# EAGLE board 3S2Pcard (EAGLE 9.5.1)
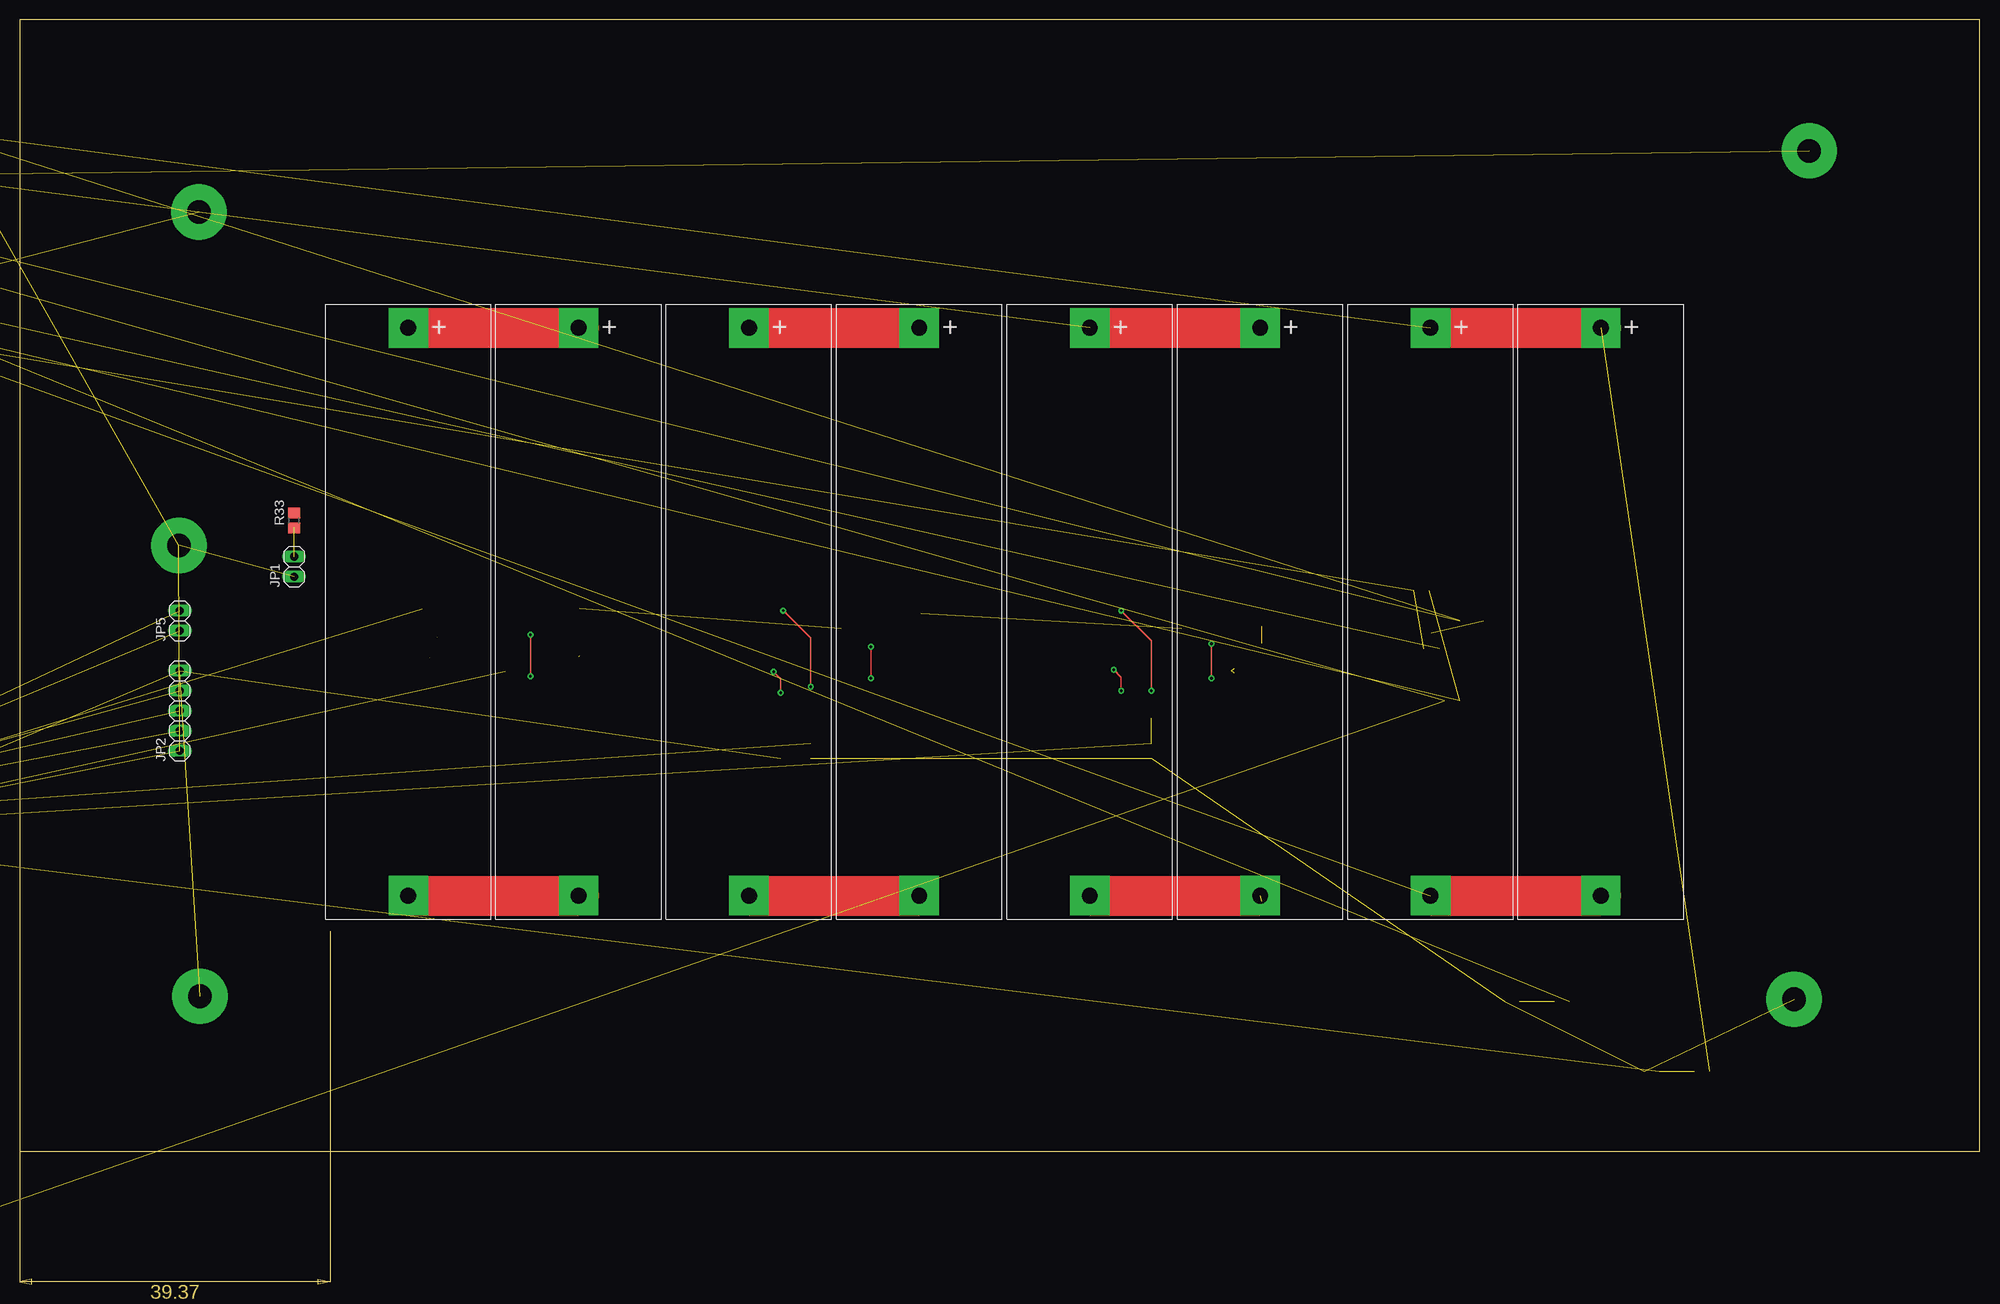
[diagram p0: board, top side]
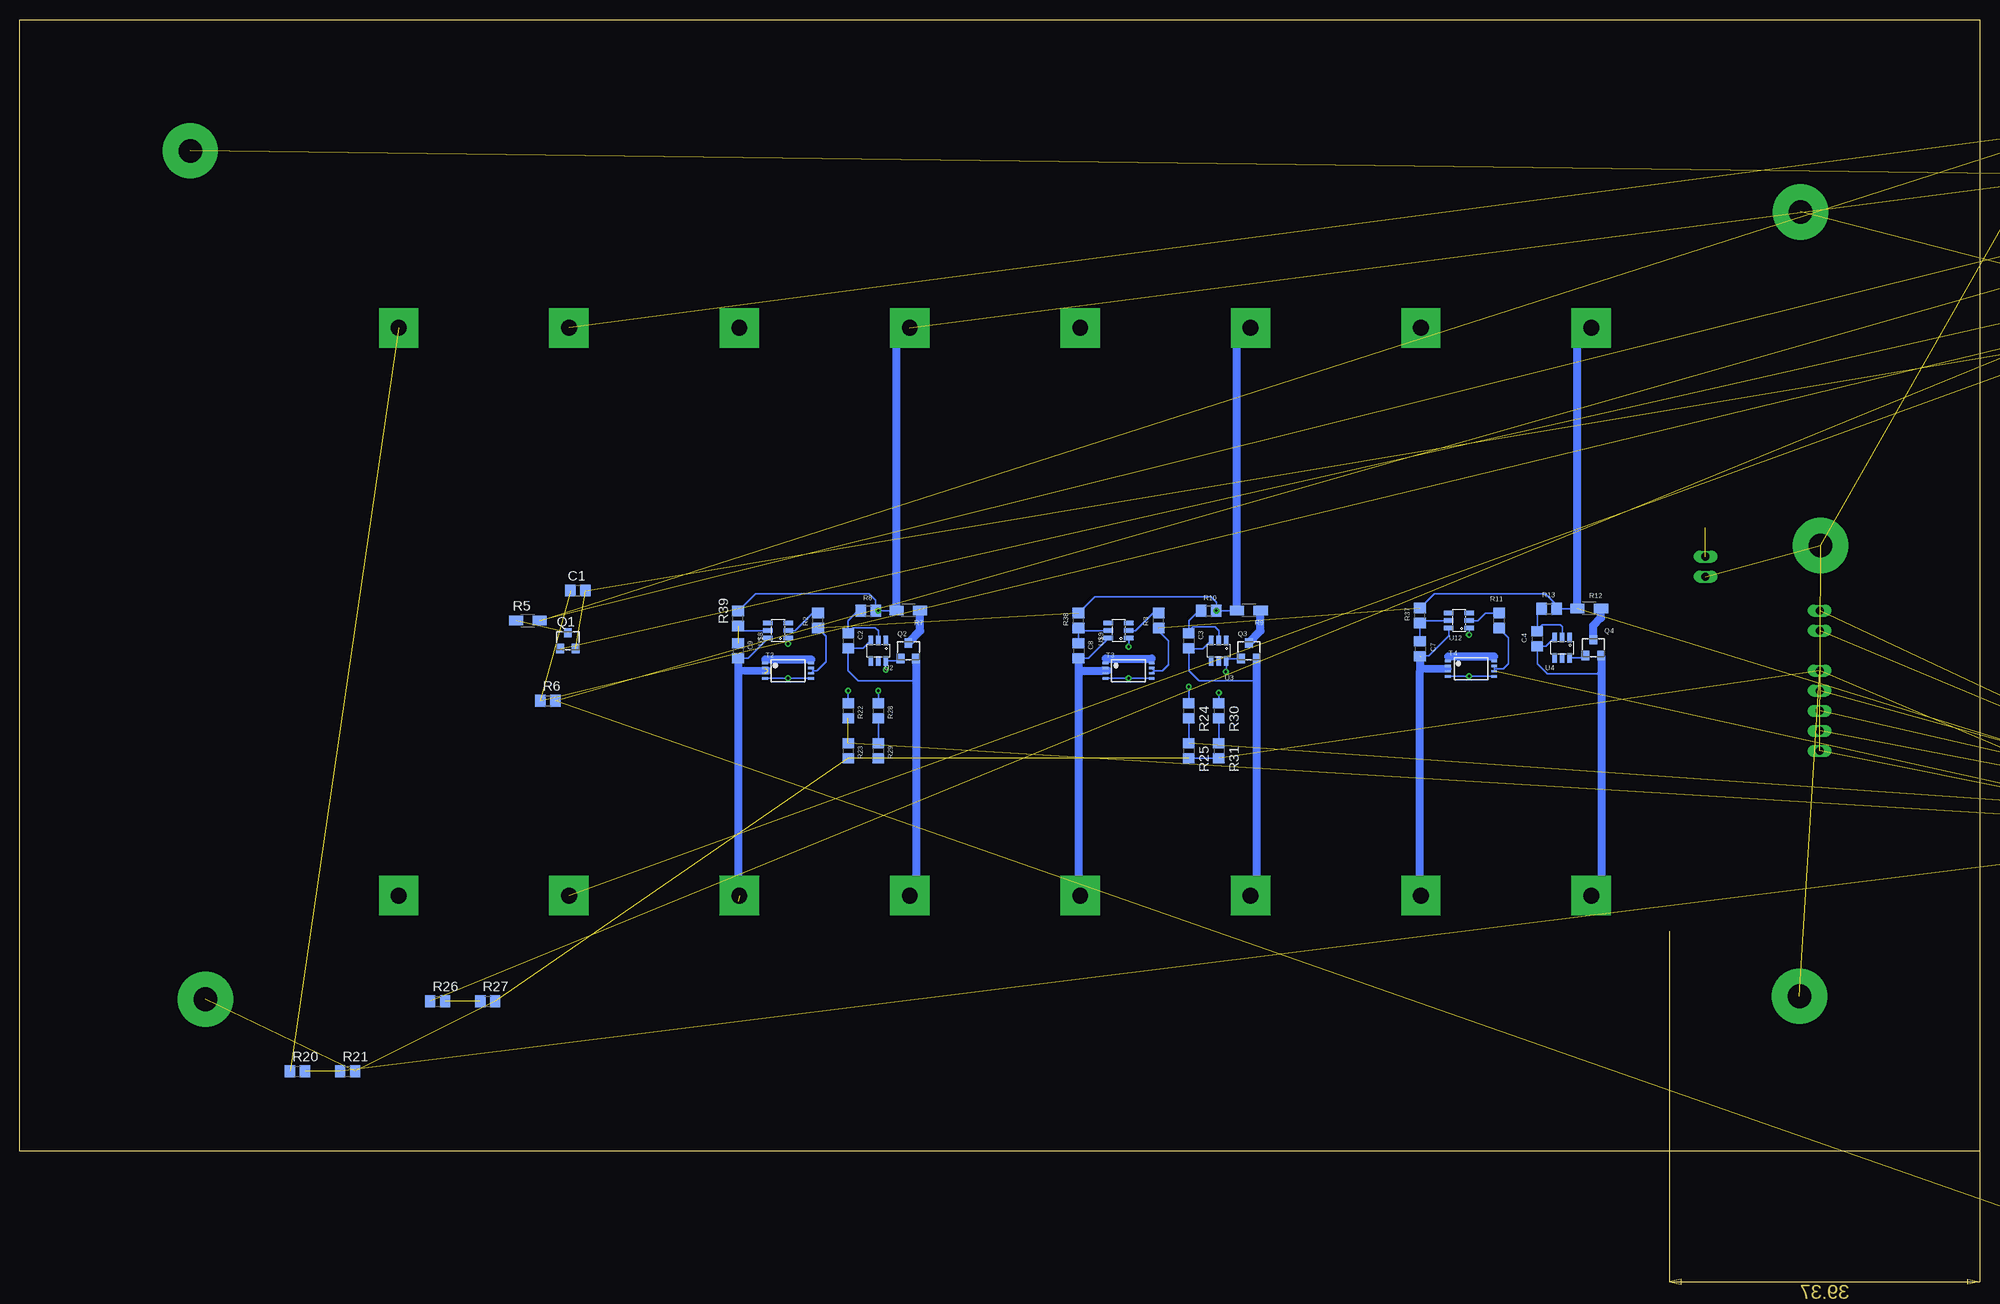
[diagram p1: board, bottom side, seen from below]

Size 248.59 x 160.31 mm. Coordinates in mm from the lower left corner, seen from the top.
Outline: 0,16.81 248.59,16.81 248.59,160.31 0,160.31 0,16.81
Copper layers (1*16): Top 0.035mm / dielectric 1.5mm / Bottom 0.035mm
Design rules "default": minimum track width 6mil, minimum drill 0.35mm, track to track 6mil, track to pad 6mil, pad to pad 6mil, via to via 6mil, smd to smd 6mil, copper to edge 40mil, drill to drill 6mil, minimum pad ring 10mil, minimum via ring 8mil, stop-mask expansion 4mil, vias tented up to drill 0mil, thermal gap 10mil

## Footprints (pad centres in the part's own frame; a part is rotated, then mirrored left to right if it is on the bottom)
18650_HOLDER = drill 2 pad 5 square: + -0.93,38.17; - -0.93,-33.83
C0805 = smd 1.3 x 1.5: 1 -0.95,0; 2 0.95,0
SO08 = smd 0.6 x 2.2: 1 -1.905,-2.6; 2 -0.635,-2.6; 3 0.635,-2.6; 4 1.905,-2.6; 5 1.905,2.6; 6 0.635,2.6; 7 -0.635,2.6; 8 -1.905,2.6
1X02 = drill 1.016 long: 1 -1.27,0; 2 1.27,0
1X05 = drill 1.016 long: 1 -5.08,0; 2 -2.54,0; 3 0,0; 4 2.54,0; 5 5.08,0
0207/10 = drill 0.813 octagon: 1 -5.08,0; 2 5.08,0
CHIP-LED0805 = smd 1.2 x 1.2: A 0,-1.05; C 0,1.05
TO236 = smd 1 x 1.2: 1 0,1; 2 -1,-1; 3 1,-1
SOIC8 = smd 0.6 x 2.2: 1 -1.905,-2.6; 2 -0.635,-2.6; 3 0.635,-2.6; 4 1.905,-2.6; 5 1.905,2.6; 6 0.635,2.6; 7 -0.635,2.6; 8 -1.905,2.6
SOT-23-CBE = smd 1 x 1.4: B -0.95,-1.1; C 0,1.1; E 0.95,-1.1
R0805 = smd 1.3 x 1.5: 1 -0.95,0; 2 0.95,0
R-27X13 = drill 1 square: 1 3.34,6.25; 2 23.66,6.25
R1206W = smd 1.8 x 1.2: 1 -1.499,0; 2 1.499,0
TSSOP-8 = smd 0.3 x 0.75: 1 -0.975,-2.925; 2 -0.325,-2.925; 3 0.325,-2.925; 4 0.975,-2.925; 5 0.975,2.925; 6 0.325,2.925; 7 -0.325,2.925; 8 -0.975,2.925
SOT23-6 = smd 0.55 x 1.2: 1 -0.95,-1.3; 2 0,-1.3; 3 0.95,-1.3; 4 0.95,1.3; 5 0,1.3; 6 -0.95,1.3
QFP80P900X900X120-32N = smd 1.473 x 0.508: 1 -4.242,2.794; 2 -4.242,2.007; 3 -4.242,1.194; 4 -4.242,0.406; 5 -4.242,-0.406; 6 -4.242,-1.194; 7 -4.242,-2.007; 8 -4.242,-2.794; 17 4.242,-2.794; 18 4.242,-2.007; 19 4.242,-1.194; 20 4.242,-0.406; 21 4.242,0.406; 22 4.242,1.194; 23 4.242,2.007; 24 4.242,2.794 | smd 0.508 x 1.473: 9 -2.794,-4.242; 10 -2.007,-4.242; 11 -1.194,-4.242; 12 -0.406,-4.242; 13 0.406,-4.242; 14 1.194,-4.242; 15 2.007,-4.242; 16 2.794,-4.242; 25 2.794,4.242; 26 2.007,4.242; 27 1.194,4.242; 28 0.406,4.242; 29 -0.406,4.242; 30 -1.194,4.242; 31 -2.007,4.242; 32 -2.794,4.242
SPACER = drill 3 pad 7: 1 0,0

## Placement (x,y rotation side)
B11  18650_HOLDER  [18650_HOLDER]  71.81,83.07 0 top
B12  18650_HOLDER  [18650_HOLDER]  50.21,83.07 0 top
B21  18650_HOLDER  [18650_HOLDER]  115.03,83.07 0 top
B22  18650_HOLDER  [18650_HOLDER]  93.42,83.07 0 top
B31  18650_HOLDER  [18650_HOLDER]  158.25,83.07 0 top
B32  18650_HOLDER  [18650_HOLDER]  136.64,83.07 0 top
B41  18650_HOLDER  [18650_HOLDER]  179.85,83.07 0 top
B42  18650_HOLDER  [18650_HOLDER]  201.46,83.07 0 top
C1  [C0805]  177.8,87.93 0 bottom
C2  [C0805]  143.51,81.58 270 bottom
C3  [C0805]  100.33,81.58 270 bottom
C4  [C0805]  56.13,81.83 270 bottom
C5  [C0805]  not placed on the board
C6  [C0805]  not placed on the board
C7  100nF  [C0805]  70.99,80.56 270 bottom
C8  100nF  [C0805]  114.3,80.31 270 bottom
C9  100nF  [C0805]  157.48,80.31 270 bottom
C10  100nF  [C0805]  not placed on the board
IC1  LM358D  [SO08]  not placed on the board
JP1  [1X02]  34.8,90.98 90 top
JP2  [1X05]  20.32,72.69 90 top
JP3  [1X02]  not placed on the board
JP4  [1X02]  not placed on the board
JP5  [1X02]  20.32,84.12 90 top
L1  [0207/10]  not placed on the board
L2  [0207/10]  not placed on the board
L3  [0207/10]  not placed on the board
LED1  RED  [CHIP-LED0805]  not placed on the board
LED2  GREEN  [CHIP-LED0805]  not placed on the board
LED3  BLUE  [CHIP-LED0805]  not placed on the board
Q1  2302  [TO236]  179.07,81.58 0 bottom
Q2  2302  [TO236]  135.89,80.31 0 bottom
Q3  2302  [TO236]  92.71,80.31 0 bottom
Q4  2302  [TO236]  49.02,80.69 0 bottom
Q5  AO4407  [SOIC8]  not placed on the board
Q6  MMBT2222  [SOT-23-CBE]  not placed on the board
Q7  AO4407  [SOIC8]  not placed on the board
Q8  MMBT2222  [SOT-23-CBE]  not placed on the board
R1  1K  [R0805]  not placed on the board
R2  1K  [R0805]  147.32,84.12 90 bottom
R3  1K  [R0805]  104.14,84.12 90 bottom
R4  R-POWER-27X13  [R-27X13]  not placed on the board
R5  [R1206W]  184.15,84.12 0 bottom
R6  [R0805]  181.61,73.96 0 bottom
R7  [R1206W]  135.89,85.39 180 bottom
R8  [R0805]  140.97,85.39 0 bottom
R9  [R1206W]  92.71,85.39 180 bottom
R10  [R0805]  97.79,85.39 0 bottom
R11  1K  [R0805]  60.96,84.12 90 bottom
R12  [R1206W]  49.53,85.64 180 bottom
R13  [R0805]  54.61,85.64 0 bottom
R14  [R0805]  not placed on the board
R15  [R0805]  not placed on the board
R16  [R0805]  not placed on the board
R17  [R0805]  not placed on the board
R18  [R0805]  not placed on the board
R19  [R0805]  not placed on the board
R20  100K  [R0805]  213.36,26.97 0 bottom
R21  470K  [R0805]  207.01,26.97 0 bottom
R22  100K  [R0805]  143.51,72.69 270 bottom
R23  330K  [R0805]  143.51,67.61 270 bottom
R24  100K  [R0805]  100.33,72.69 270 bottom
R25  220K  [R0805]  100.33,67.61 270 bottom
R26  100K  [R0805]  195.58,35.86 0 bottom
R27  470K  [R0805]  189.23,35.86 0 bottom
R28  100K  [R0805]  139.7,72.69 270 bottom
R29  330K  [R0805]  139.7,67.61 270 bottom
R30  100K  [R0805]  96.52,72.69 270 bottom
R31  220K  [R0805]  96.52,67.61 270 bottom
R32  [R0805]  not placed on the board
R33  330K  [R0805]  34.8,96.82 90 top
R34  1K  [R0805]  not placed on the board
R35  1K  [R0805]  not placed on the board
R36  1K  [R0805]  not placed on the board
R37  100E  [R0805]  70.99,84.75 90 bottom
R38  100E  [R0805]  114.3,84.12 90 bottom
R39  100E  [R0805]  157.48,84.37 90 bottom
R40  100E  [R0805]  not placed on the board
T1  DMN3024LSD  [TSSOP-8]  not placed on the board
T2  DMN3024LSD  [TSSOP-8]  151.13,77.77 270 bottom
T3  DMN3024LSD  [TSSOP-8]  107.95,77.77 270 bottom
T4  DMN3024LSD  [TSSOP-8]  64.52,78.02 270 bottom
U1  HY2213  [SOT23-6]  not placed on the board
U2  HY2213  [SOT23-6]  139.7,80.31 180 bottom
U3  HY2213  [SOT23-6]  96.52,80.31 180 bottom
U4  HY2213  [SOT23-6]  52.96,80.69 180 bottom
U5  ATMEGA328P-AU  [QFP80P900X900X120-32N]  not placed on the board
U12  DW01A  [SOT23-6]  66.04,84.12 90 bottom
U$7  DW01A  [SOT23-6]  not placed on the board
U$8  DW01A  [SOT23-6]  152.4,82.85 90 bottom
U$9  DW01A  [SOT23-6]  109.22,82.85 90 bottom
U$13  METAL_SPACER  [SPACER]  226.95,143.68 0 top
U$14  METAL_SPACER  [SPACER]  225.04,36.11 0 top
U$15  METAL_SPACER  [SPACER]  22.73,135.94 0 top
U$16  METAL_SPACER  [SPACER]  22.86,36.5 0 top
U$17  METAL_SPACER  [SPACER]  20.19,93.64 0 top

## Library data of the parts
B11 B12 B21 B22 B31 B32 B41 B42 U$13-U$17 = drag-custom
C1-C10 = rcl; SPICEPREFIX: C
IC1 = linear
JP1-JP5 = pinhead
L1-L3 = rcl; SPICEPREFIX: L
LED1-LED3 = led
Q1-Q8 U1-U4 = drag-semiconductors
R1-R3 R5-R40 = rcl; SPICEPREFIX: R
R4 = drag-rlcd
T1-T4 = FS8205A
U5 = ATmega328-AU; DESCRIPTION: 8-bit Microcontroller with In-System Programmable Flash; MPN: ATMEGA328P-AU; OC_FARNELL: 1715486; OC_NEWARK: 14R4631; PACKAGE: TQFP-32; SUPPLIER: Atmel
U12 U$7-U$9 = DW01A

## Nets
1S+: B11.+ B12.+ R3.1 R12.2 R13.2 R37.2 T3.6 T3.7 U5.26
1S-: B11.- B12.- C4.2 C7.2 Q4.3 T4.2 T4.3 U4.3 U12.6
1S_STATUS: Q4.2 U4.6
2S+: B21.+ B22.+ R2.1 R9.2 R10.2 R24.1 R38.2 T2.6 T2.7
2S-: B21.- B22.- C3.2 C8.2 Q3.3 T3.2 T3.3 U3.3 U$9.6
2S_STATUS: R30.2 R31.1
3S+: B31.+ B32.+ R1.1 R7.2 R8.2 R22.1 R39.2 T1.6 T1.7
3S-: B31.- B32.- C2.2 C9.2 Q2.3 T2.2 T2.3 U2.3 U$8.6
3S_STATUS: R28.2 R29.1
4S+: B41.+ B42.+ JP4.1 L1.2 Q7.5 Q7.6 Q7.7 Q7.8 R5.2 R6.2 R18.2 R20.1 R40.2
4S-: B41.- B42.- C1.2 C10.2 Q1.3 T1.2 T1.3 U1.3 U$7.6
4S_STATUS: R26.2 R27.1
5V: IC1.8 JP1.1 JP2.1 L3.1 LED1.A LED2.A LED3.A R15.2 U5.4 U5.6 U$17.1
ADC_2S: R24.2 R25.1 U5.25
ADC_3S: R22.2 R23.1 U5.24
ADC_4S: R20.2 R21.1 U5.23
BATT_CURR: C5.1 IC1.1 IC1.2 R14.2 R15.1 R32.1 R32.2
CH_SWITCH: R17.2
CHARGE+: JP3.1 Q5.5 Q5.6 Q5.7 Q5.8 R16.2 U$15.1
GND: C5.2 C6.2 IC1.4 JP2.5 Q6.E Q8.E R4.1 R14.1 R21.2 R23.2 R25.2 R27.2 R29.2 R31.2 U5.3 U5.5 U5.21 U$14.1 U$16.1
LOAD+: L2.2 U$13.1
LOAD_SWITCH: R19.2
N$1: C7.1 R37.1 U12.5
N$2: T1.1 T1.8
N$3: C8.1 R38.1 U$9.5
N$5: T2.1 T2.8
N$6: R33.2
N$7: C9.1 R39.1 U$8.5
N$8: C10.1 R40.1 U$7.5
N$9: R1.2 U$7.2
N$10: T1.4 T1.5 U$7.1
N$11: R2.2 U$8.2
N$12: T3.1 T3.8
N$13: C6.1 L3.2 U5.18
N$14: T2.4 T2.5 U$8.1
N$15: LED1.C R34.1
N$16: LED2.C R35.1
N$17: T3.4 T3.5 U$9.1
N$18: R3.2 U$9.2
N$19: LED3.C R36.1
N$20: C1.1 R6.1 U1.2
N$22: Q1.2 R26.1 U1.6
N$23: Q1.1 R5.1
N$25: C2.1 R8.1 U2.2
N$26: Q2.2 R28.1 U2.6
N$27: Q2.1 R7.1
N$28: JP3.2 L1.1 Q5.1 Q5.2 Q5.3
N$30: C3.1 R10.1 U3.2
N$31: Q3.2 R30.1 U3.6
N$32: Q3.1 R9.1
N$33: T4.1 T4.8
N$34: T4.4 T4.5 U12.1
N$36: R11.2 U12.2
N$37: C4.1 R13.1 U4.2
N$38: JP4.2
N$39: Q4.1 R12.1
N$40: IC1.3 R4.2 R11.1 T4.6 T4.7
N$41: Q5.4 Q6.C R16.1
N$42: Q6.B R17.1
N$46: L2.1 Q7.1 Q7.2 Q7.3
N$47: Q7.4 Q8.C R18.1
N$48: Q8.B R19.1
RST: JP2.2 U5.29
RX: JP2.4 U5.30
SCL: JP5.1 U5.28
SDA: JP5.2 U5.27
THERM_ADC: JP1.2 R33.1
TX: JP2.3 U5.31

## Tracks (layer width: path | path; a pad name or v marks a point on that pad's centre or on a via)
1S+  (2 unrouted)
  Top 5.08: B12.+ B11.+
  Bottom 0.203: R12.2 R13.2 53.66,86.09 55.12,87.55 69.15,87.55 R37.2 | R3.1 104.14,82.85 102.87,81.58 102.87,78.53 103.63,77.77 104.7,77.77 | 104.7,77.77 T3.7 | 104.7,77.77 T3.6
  Bottom 1.016: R12.2 51.03,119.49 B12.+
1S-  (1 unrouted)
  Top 5.08: B12.- B11.-
  Bottom 0.203: T4.2 67.44,78.02 T4.3 | 70.9,79.52 71.02,79.64 | 71.02,79.64 71.18,79.8 | U4.3 55.02,80.88 C4.2 56.13,78.66 54.86,77.39 48.02,77.39 | U12.6 67.34,82.19 69.88,79.64 71.02,79.64
  Bottom 0.94: 70.99,77.77 70.74,78.02 67.44,78.02
  Bottom 1.016: B12.- 48.02,50.49 48.02,77.39 Q4.3 | C7.2 70.99,77.77 70.99,49.35 B11.-
1S_STATUS  (1 unrouted)
  Bottom 0.203: Q4.2 50.28,79.44 51.96,79.44 U4.6
2S+  (via drill 0.35)  (1 unrouted)
  Top 0.203: v100.33,75.74 100.33,81.96 96.9,85.39 R10.2
  Top 5.08: B22.+ B21.+
  Bottom 0.203: R9.2 R10.2 96.84,86.47 97.54,87.17 112.2,87.17 R38.2 | R24.1 v100.33,75.74 | R2.1 146.3,82.15 146.3,78.91 147.45,77.77 147.88,77.77 | T2.7 147.88,77.77 | 147.88,77.77 T2.6
  Bottom 1.016: R9.2 94.21,119.52 B22.+
  other vias: 96.84,85.39
2S-
  Top 5.08: B22.- B21.-
  Bottom 0.203: U3.3 98.52,80.56 100.26,80.56 | 100.26,80.56 C3.2 | 91.71,76.5 99.06,76.5 100.33,77.77 100.33,80.5 100.26,80.56 | U$9.6 113.06,79.36 C8.2 | 111.2,77.77 T3.2 | 111.25,77.77 111.2,77.77 | 111.2,77.77 T3.3
  Bottom 0.889: 111.25,77.77 110.49,77.77
  Bottom 1.016: Q3.3 91.71,76.5 91.71,50.02 B22.- | C8.2 114.3,77.77 | 114.3,77.77 114.3,49.44 B21.- | 114.3,77.77 111.25,77.77
2S_STATUS
  Bottom 0.203: R30.2 R31.1
3S+  (via drill 0.35)  (3 unrouted)
  Top 0.203: v143.51,75.23 143.51,81.58 v139.7,85.39
  Top 5.08: B32.+ B31.+
  Bottom 0.203: R7.2 v139.7,85.39 R8.2 140.02,86.73 140.84,87.55 155.25,87.55 R39.2 | R22.1 v143.51,75.23
  Bottom 1.016: R7.2 137.39,119.56 B32.+
3S-  (3 unrouted)
  Top 5.08: B32.- B31.-
  Bottom 0.203: U2.3 141.63,80.63 C2.2 143.51,77.77 142.24,76.5 134.89,76.5 | U$8.6 156.24,79.36 C9.2
  Bottom 0.94: 157.48,77.77 153.67,77.77
  Bottom 1.016: Q2.3 134.89,76.5 134.89,50.06 B32.- | C9.2 157.48,77.77 157.48,48.56
3S_STATUS
  Bottom 0.203: R29.1 R28.2
4S+  (11 unrouted)
  Top 5.08: B41.+ B42.+
4S-  (7 unrouted)
  Top 5.08: B41.- B42.-
4S_STATUS  (1 unrouted)
5V  (10 unrouted)
ADC_2S  (1 unrouted)
  Bottom 0.203: R24.2 R25.1
ADC_3S  (2 unrouted)
ADC_4S  (2 unrouted)
BATT_CURR  (6 unrouted)
CHARGE+  (6 unrouted)
GND  (17 unrouted)
  Bottom 0.203: R31.2 R25.2
LOAD+  (1 unrouted)
N$1
  Bottom 0.203: C7.1 R37.1 70.68,84.12 U12.5
N$2  (1 unrouted)
N$3
  Bottom 0.203: R38.1 114.3,82.85 | 114.3,82.85 C8.1 | U$9.5 114.3,82.85
N$5
  Bottom 0.203: T2.8 148.21,79.04 | 148.21,79.04 148.21,79.29 | T2.1 154.06,79.17 154.06,79.29 154.05,79.29 | 148.21,79.04 148.21,79.17
  Bottom 1.016: 148.21,79.17 154.06,79.17
N$7  (1 unrouted)
  Bottom 0.203: U$8.5 157.1,82.85 157.48,83.23 R39.1
N$8  (2 unrouted)
N$9  (1 unrouted)
N$10  (2 unrouted)
N$11
  Bottom 0.203: R2.2 148.02,85.07 150.24,82.85 U$8.2
N$12
  Bottom 0.203: T3.8 105.03,79.29 | T3.1 110.88,79.29 110.87,79.29
  Bottom 1.016: 110.87,79.29 105.03,79.29
N$13  (2 unrouted)
N$14  (via drill 0.35)
  Top 0.203: v151.13,81.2 v151.13,76.8
  Bottom 0.203: T2.5 v151.13,76.8 T2.4 | U$8.1 151.1,81.23 v151.13,81.2
N$15  (1 unrouted)
N$16  (1 unrouted)
N$17  (via drill 0.35)
  Top 0.203: v107.95,80.82 v107.95,76.8
  Bottom 0.203: T3.5 v107.95,76.8 T3.4 | U$9.1 107.92,80.85 v107.95,80.82
N$18
  Bottom 0.203: R3.2 104.84,85.07 107.06,82.85 U$9.2
N$19  (1 unrouted)
N$20  (2 unrouted)
N$22  (2 unrouted)
N$23  (1 unrouted)
N$25
  Bottom 0.203: R8.1 142.24,85.39 143.51,84.12 C2.1 143.51,82.6 142.88,83.23 140.08,83.23 139.7,82.85 U2.2
N$26  (via drill 0.35)
  Top 0.203: v138.75,77.9 139.7,76.95 v139.7,75.23
  Bottom 0.203: Q2.2 137.19,79.01 U2.6 v138.75,77.9 | v139.7,75.23 R28.1
N$27
  Bottom 1.016: Q2.1 134.39,82.81 R7.1
N$28  (4 unrouted)
N$30
  Bottom 0.203: R10.1 99.06,85.39 100.33,84.12 100.33,82.85 | 100.33,82.85 C3.1 | U3.2 96.52,82.85 97.03,83.36 99.82,83.36 100.33,82.85
N$31  (via drill 0.35)
  Top 0.203: v96.52,74.98 96.52,76.75 v95.63,77.64
  Bottom 0.203: R30.1 v96.52,74.98 | v95.63,77.64 95.57,77.7 U3.6 95.27,79.31 Q3.2
N$32
  Bottom 1.016: Q3.1 91.21,82.81 R9.1
N$33
  Bottom 0.203: T4.8 61.59,79.54 | T4.1 67.44,79.54
  Bottom 0.356: 61.59,79.54 61.59,79.55 | 67.44,79.54 67.44,79.55
  Bottom 1.016: 61.59,79.54 67.44,79.54
N$34  (via drill 0.35)
  Top 0.203: v64.77,82.34 v64.77,77.05
  Bottom 0.203: T4.5 v64.77,77.05 T4.4 | U12.1 64.74,82.37 v64.77,82.34
N$36
  Bottom 0.203: U12.2 63.63,84.12 62.68,85.07 R11.2
N$37  (1 unrouted)
  Bottom 0.203: 52.99,81.99 U4.2 52.96,83.36 53.21,83.61 55.5,83.61 56.13,82.98 | C4.1 56.13,82.98 | 56.13,82.98 56.13,85.07 R13.1
N$39
  Bottom 1.016: Q4.1 49.02,83.48 48.03,84.48 R12.1
N$40  (2 unrouted)
  Bottom 0.203: T4.7 61.59,78.02 | 61.59,78.02 T4.6 | R11.1 60.96,83.1 | 60.96,83.1 60.96,82.6 | 61.59,78.02 60.45,78.02 59.82,78.66 59.82,81.96 60.96,83.1
N$41  (2 unrouted)
N$42  (1 unrouted)
N$46  (3 unrouted)
N$47  (2 unrouted)
N$48  (1 unrouted)
RST  (1 unrouted)
RX  (1 unrouted)
SCL  (1 unrouted)
SDA  (1 unrouted)
THERM_ADC  (1 unrouted)
TX  (1 unrouted)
